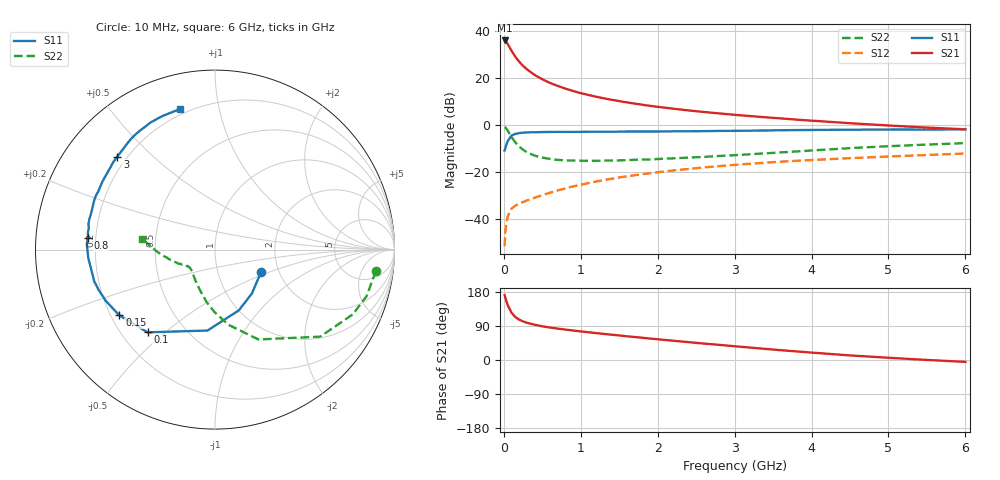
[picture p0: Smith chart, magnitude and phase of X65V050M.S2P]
! SIEMENS Small Signal Semiconductors
! BFP193W
! Si NPN RF Bipolar Junction Transistor in SOT343
! VCE = 5 V  IC = 50 mA
! Common Emitter S-Parameters:  April 1994
# GHz  S  MA  R  50
!  f  S11  S21  S12  S22
! GHz  MAG  ANG  MAG  ANG  MAG  ANG  MAG  ANG
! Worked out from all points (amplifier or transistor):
!   40 points, 10 MHz to 6 GHz, reference 50 ohm
!   highest |S21| = 36.1 dB at 10 MHz (marker M1)
!   |S21| within 3 dB of that: start of sweep to 75.72 MHz
!   unconditionally stable (mu >= 1): 649.5 MHz to 4.132 GHz
!   at 200 MHz: K = 0.56, MSG = 30.2 dB, |S12| = -33.5 dB
!   at 1.5 GHz: K = 1.12, MAG = 14.2 dB, |S12| = -22.4 dB
!   at 6 GHz: K = 0.95, MSG = 5.2 dB, |S12| = -12.2 dB
!   S11 on the Smith chart (normalised r, x): 10 MHz: 1.61, -0.45; 100 MHz: 0.31, -0.44; 150 MHz: 0.23, -0.29; 800 MHz: 0.17, +0.04; 3 GHz: 0.16, +0.39; 6 GHz: 0.17, +0.77
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0.01  0.2856 -26.5  63.67 171.2  0.0026 83.9  0.904 -7.6
0.02  0.3198 -50.1  62.19 164.4  0.0054 73.1  0.8836 -17.1
0.03  0.3638 -68.7  59.97 157.3  0.0073 72.5  0.8479 -25.2
0.05  0.4529 -95.3  53.44 144.9  0.0112 63.1  0.7609 -39.6
0.1  0.5947 -129.2  38.39 124.8  0.0165 49.2  0.556 -64.2
0.15  0.6467 -145.5  28.54 113.2  0.019 45.4  0.4253 -79.9
0.2  0.6719 -154.8  22.33 106.5  0.0211 45.8  0.3463 -90.7
0.25  0.6861 -160.8  18.33 101.8  0.0227 46.5  0.2975 -98.8
0.3  0.6957 -165.2  15.4 98.2  0.0246 48.0  0.2611 -105.6
0.4  0.6993 -171.6  11.71 93.0  0.0281 51.1  0.2225 -115.6
0.5  0.7075 -176.1  9.456 88.9  0.0319 54.7  0.2017 -123.2
0.6  0.7107 -179.6  7.898 85.6  0.0359 56.6  0.1886 -129.1
0.8  0.7109 174.9  5.967 80.3  0.0444 59.7  0.1757 -136.4
1.1  0.7195 168.5  4.376 73.2  0.0577 61.5  0.1718 -143.4
1.3  0.7191 164.3  3.705 68.8  0.0669 62.0  0.1739 -145.8
1.6  0.7252 158.9  3.037 62.6  0.0805 61.4  0.1776 -148.6
2.2  0.7328 148.9  2.232 50.9  0.107 58.5  0.1943 -154.1
3  0.7519 136.4  1.65 36.3  0.1411 52.9  0.2267 -161.6
3.2  0.7569 133.4  1.554 32.8  0.1489 51.5  0.238 -163.4
4.5  0.7944 116.6  1.093 12.1  0.1961 41.7  0.3214 -177.7
5.5  0.8013 108.1  0.882 0.2  0.2294 35.0  0.3823 174.4
6  0.8076 103.9  0.81 -5.0  0.2465 32.0  0.4114 171.5
